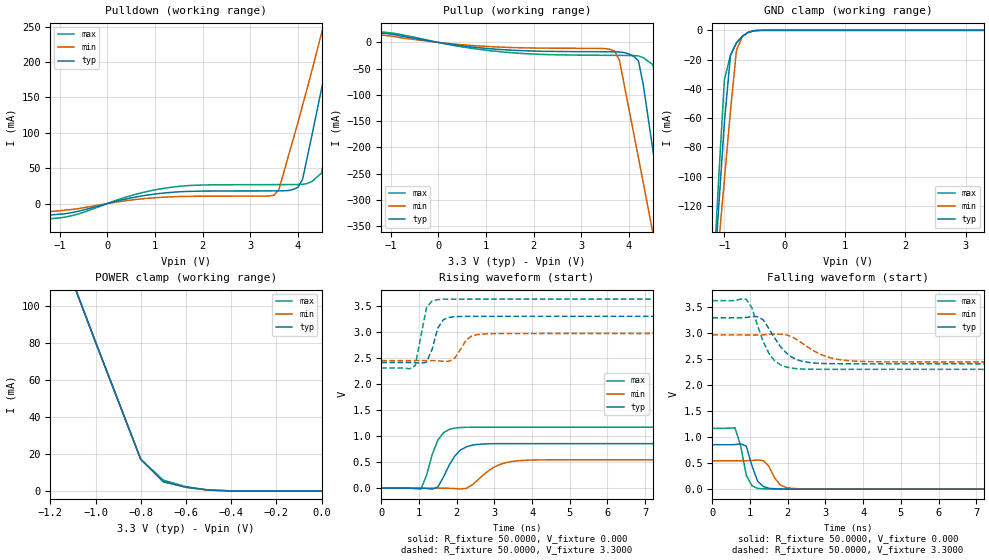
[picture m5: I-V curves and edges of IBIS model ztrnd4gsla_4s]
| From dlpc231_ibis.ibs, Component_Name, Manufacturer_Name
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| Model ztrnd4gsla_4s
[Model]   ztrnd4gsla_4s
Model_type   I/O
Polarity   Non-Inverting
Enable   Active-High
Vinl = 0.8000V
Vinh = 2.0000V
Vmeas = 1.5000V
Cref =50.0000pF
Rref = 0.5000k
Vref =  0.000V
C_comp   0.7000pF   0.7000pF   0.7000pF
[Temperature Range]   25.0000   0.1240k   -40.0000
[Voltage Range]   3.3000V   2.9700V   3.6300V
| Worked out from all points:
|   slope of the pulldown table from 0 to 0.495 V, typ, clamps not added: 62.5 ohm
|   slope of the pullup table from 0 to 0.495 V, typ, clamps not added: 77 ohm
|   GND clamp passes 1 mA (typ) near -0.57 V on its own axis
|   POWER clamp passes 1 mA (typ) near -0.54 V on its own axis
|   rising waveform, R_fixture 50.0000, V_fixture 0.000: 20-80 % time 421ps typ, 606ps min, 321ps max; typ from 0 V to 0.856 V
|   rising waveform, R_fixture 50.0000, V_fixture 3.3000: 20-80 % time 242ps typ, 296ps min, 214ps max; typ from 2.41 V to 3.3 V
|   falling waveform, R_fixture 50.0000, V_fixture 0.000: 20-80 % time 233ps typ, 265ps min, 219ps max; typ from 0.856 V to 0 V
|   falling waveform, R_fixture 50.0000, V_fixture 3.3000: 20-80 % time 547ps typ, 761ps min, 441ps max; typ from 3.3 V to 2.41 V
[Pulldown]
-3.3V     -24mA      -18mA      -30mA
-900mV    -14.55mA   -9.41mA    -19.37mA
1.4V      16.11mA    9.655mA    23.49mA
3.5V      17.9mA     11.77mA    26.76mA
3.6V      17.91mA    19.43mA    26.77mA
3.9V      19.9mA     90.39mA    26.83mA
4.1V      34.51mA    138.9mA    27.06mA
4.5V      163.1mA    241.5mA    43.23mA
4.7V      230.5mA    296.1mA    120.2mA
4.9V      300.3mA    353.6mA    204.3mA
5.1V      373.1mA    414.8mA    291.1mA
6.6V      1.049A     968.2mA    1.056A
[Pullup]
-3.3V     15mA       18.5mA     10mA
-1.5V     21.2mA     17.2mA     22.7mA
1.2V      -12.77mA   -8.444mA   -16.81mA
3.7V      -17.91mA   -16.46mA   -24.61mA
3.8V      -18.14mA   -33.44mA   -24.66mA
4.2V      -34.83mA   -219.7mA   -25.74mA
4.3V      -79.52mA   -266.7mA   -28.82mA
4.5V      -202.8mA   -361.2mA   -42.15mA
4.7V      -327.1mA   -456.4mA   -104.6mA
4.9V      -452.4mA   -552.1mA   -260.7mA
5.1V      -578.3mA   -648.3mA   -417.9mA
6.6V      -1.534A    -1.38A     -1.61A
[GND_clamp]
-3.3V     -1.517A    -1.206A    -1.849A
-1.2V     -185.7mA   -194.8mA   -182.8mA
-1.1V     -124mA     -148.1mA   -104.8mA
-1V       -62.54mA   -101.7mA   -33.61mA
-900mV    -17.04mA   -55.16mA   -17.04mA
-800mV    -8.525mA   -13.45mA   -8.525mA
-700mV    -3.999mA   -3.999mA   -3.999mA
-600mV    -1.289mA   -1.289mA   -1.289mA
-500mV    -219.7uA   -252.6uA   -203.6uA
-400mV    -15.61uA   -27.49uA   -11.15uA
3.3V      3.373nA    3.373nA    17.05nA
[POWER_clamp]
-3.3V     1.027A     840.1mA    1.22A
-1.1V     112.7mA    112.7mA    112.7mA
-1V       80.41mA    80.41mA    80.41mA
-800mV    17.08mA    17.08mA    17.08mA
-700mV    4.947mA    4.947mA    5.794mA
-600mV    1.98mA     1.98mA     2.27mA
-500mV    443.8uA    443.8uA    443.8uA
-400mV    34.78uA    34.78uA    34.78uA
0V        3.373nA    3.373nA    57.43nA
[Ramp]
dV/dt_r   0.5134/0.4086n   0.3275/0.5915n   0.7026/0.3160n
dV/dt_f   0.5322/0.5362n   0.3126/0.7568n   0.7938/0.4331n
R_load = 50.0000
[Rising Waveform]
R_fixture = 50.0000
V_fixture = 0.000
V_fixture_min = 0.000
V_fixture_max = 0.000
0s        0V         0V         0V
1.05ns    1.156mV    -6.408uV   -17.54mV
1.2ns     -4.694mV   -8.21uV    248.6mV
1.5ns     23.18mV    467.9uV    924.9mV
1.65ns    215.3mV    880.2uV    1.065V
1.95ns    618.4mV    -6.981mV   1.155V
2.4ns     825.5mV    58.19mV    1.17V
3ns       853.8mV    407.8mV    1.171V
3.75ns    855.6mV    532.9mV    1.171V
14.85ns   855.7mV    545.9mV    1.171V
[Rising Waveform]
R_fixture = 50.0000
V_fixture = 3.3000
V_fixture_min = 2.9700
V_fixture_max = 3.6300
0s        2.413V     2.449V     2.307V
900ps     2.412V     2.449V     2.354V
1.2ns     2.42V      2.449V     3.47V
1.35ns    2.671V     2.449V     3.595V
1.5ns     3.076V     2.446V     3.62V
1.8ns     3.279V     2.436V     3.629V
1.95ns    3.292V     2.499V     3.629V
2.25ns    3.298V     2.842V     3.63V
2.7ns     3.299V     2.959V     3.63V
14.85ns   3.3V       2.97V      3.63V
[Falling Waveform]
R_fixture = 50.0000
V_fixture = 0.000
V_fixture_min = 0.000
V_fixture_max = 0.000
0s        855.7mV    545.9mV    1.171V
600ps     859.3mV    545.7mV    1.181V
750ps     872.8mV    545.5mV    837.2mV
900ps     827.8mV    546.9mV    268.7mV
1.05ns    455.4mV    552.9mV    66.51mV
1.2ns     152.8mV    562mV      14.78mV
1.5ns     16.91mV    444.2mV    3.613mV
1.8ns     4.81mV     81.32mV    1.011mV
2.25ns    1.163mV    8.662mV    142.6uV
14.85ns   0V         0V         0V
[Falling Waveform]
R_fixture = 50.0000
V_fixture = 3.3000
V_fixture_min = 2.9700
V_fixture_max = 3.6300
0s        3.3V       2.97V      3.63V
900ps     3.307V     2.969V     3.658V
1.05ns    3.326V     2.969V     3.492V
1.2ns     3.321V     2.969V     3.147V
1.5ns     3.093V     2.981V     2.615V
1.8ns     2.752V     2.985V     2.397V
2.1ns     2.545V     2.939V     2.331V
2.85ns    2.422V     2.603V     2.308V
3.75ns    2.413V     2.466V     2.307V
14.85ns   2.413V     2.449V     2.307V
